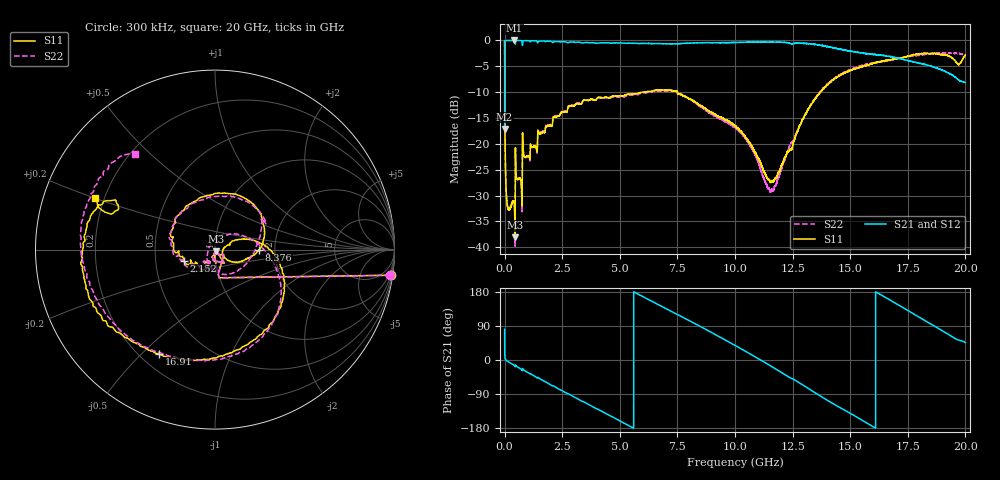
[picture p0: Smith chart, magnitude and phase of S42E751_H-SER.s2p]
! Created Wed Nov 25 22:26:33 2020
# khz S ma R 50
! 2 Port Network Data from SP1.SP block
! freq  magS11  angS11  magS21  angS21  magS12  angS12  magS22  angS22
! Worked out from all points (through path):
!   20001 points, 300 kHz to 20 GHz, reference 50 ohm
!   highest |S21| = 0.00 dB at 417.3 MHz (marker M1); lowest = -17.1 dB at 300 kHz (marker M2)
!   group delay of S21, straight-line fit = 94.2 ps
!   lowest |S11| = -38.1 dB at 454.3 MHz (marker M3), VSWR 1.03, Z = 50.7 - j1.02 ohm
!   |S11| at or under -10 dB: 6.399 MHz to 6.053 GHz (6.047 GHz wide, 200 % of centre); 6.053517 GHz to 6.058976 GHz (5.459 MHz wide, 0.0901 % of centre); 7.5 GHz to 13.7 GHz (6.204 GHz wide, 58.5 % of centre)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
!   |S22| runs from -39.8 to -0.1 dB; largest |S21 - S12| = 0.02
!   S11 on the Smith chart (normalised r, x): 300 kHz: 1, -14; 2.152 GHz: 0.70, -0.09; 8.376 GHz: 1.65, -0.01; 16.91 GHz: 0.27, -0.56; 20 GHz: 0.16, +0.20
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300  0.99 -8.3  0.1391 81.2  0.1399 81.7  0.9871 -8.4
101300  0.02731 -94.2  0.9981 -2.2  0.9991 -2.2  0.02752 -93.8
135300  0.02421 -95.7  0.9988 -3.6  0.9989 -3.6  0.02444 -95.5
417300  0.02657 -103.3  0.9996 -13.9  0.999 -14.0  0.0264 -105.0
454300  0.01247 -53.9  0.9905 -16.5  0.9905 -16.5  0.01027 -56.6
868300  0.07526 -117.2  0.9954 -27.8  0.9953 -27.8  0.07471 -118.7
2152300  0.1824 -160.3  0.9728 -69.4  0.9735 -69.4  0.1855 -154.6
3334300  0.2435 163.5  0.9495 -108.2  0.949 -108.2  0.2455 167.4
5074300  0.2915 112.3  0.9444 -163.0  0.9448 -163.1  0.2859 104.2
6667300  0.3297 64.7  0.9327 146.2  0.9307 146.1  0.3232 50.3
8376300  0.2449 -0.7  0.9482 92.3  0.9447 92.4  0.2398 7.9
1.00003e7  0.1503 -27.6  0.9556 38.5  0.9564 38.6  0.1436 -74.1
1.08413e7  0.0844 -40.2  0.9631 9.4  0.9633 9.5  0.08007 -119.0
1.16003e7  0.04392 -9.8  0.9641 -17.5  0.9649 -17.5  0.03619 150.1
1.23133e7  0.08483 18.8  0.9487 -44.2  0.951 -44.2  0.08888 65.2
1.33343e7  0.2444 9.9  0.9219 -81.0  0.9225 -80.8  0.2456 6.5
1.51093e7  0.5234 -55.2  0.7825 -144.8  0.7814 -144.9  0.5355 -56.3
1.66673e7  0.6433 -110.2  0.7031 160.6  0.689 160.5  0.6389 -109.8
1.69143e7  0.6603 -118.3  0.6861 151.6  0.6714 151.7  0.6535 -119.4
1.85163e7  0.7469 -168.9  0.5625 94.4  0.5652 95.0  0.7456 179.6
1.93993e7  0.6843 158.6  0.4669 62.3  0.4724 62.2  0.754 151.1
2e7  0.727 156.7  0.3916 46.1  0.3919 46.9  0.6884 129.7
